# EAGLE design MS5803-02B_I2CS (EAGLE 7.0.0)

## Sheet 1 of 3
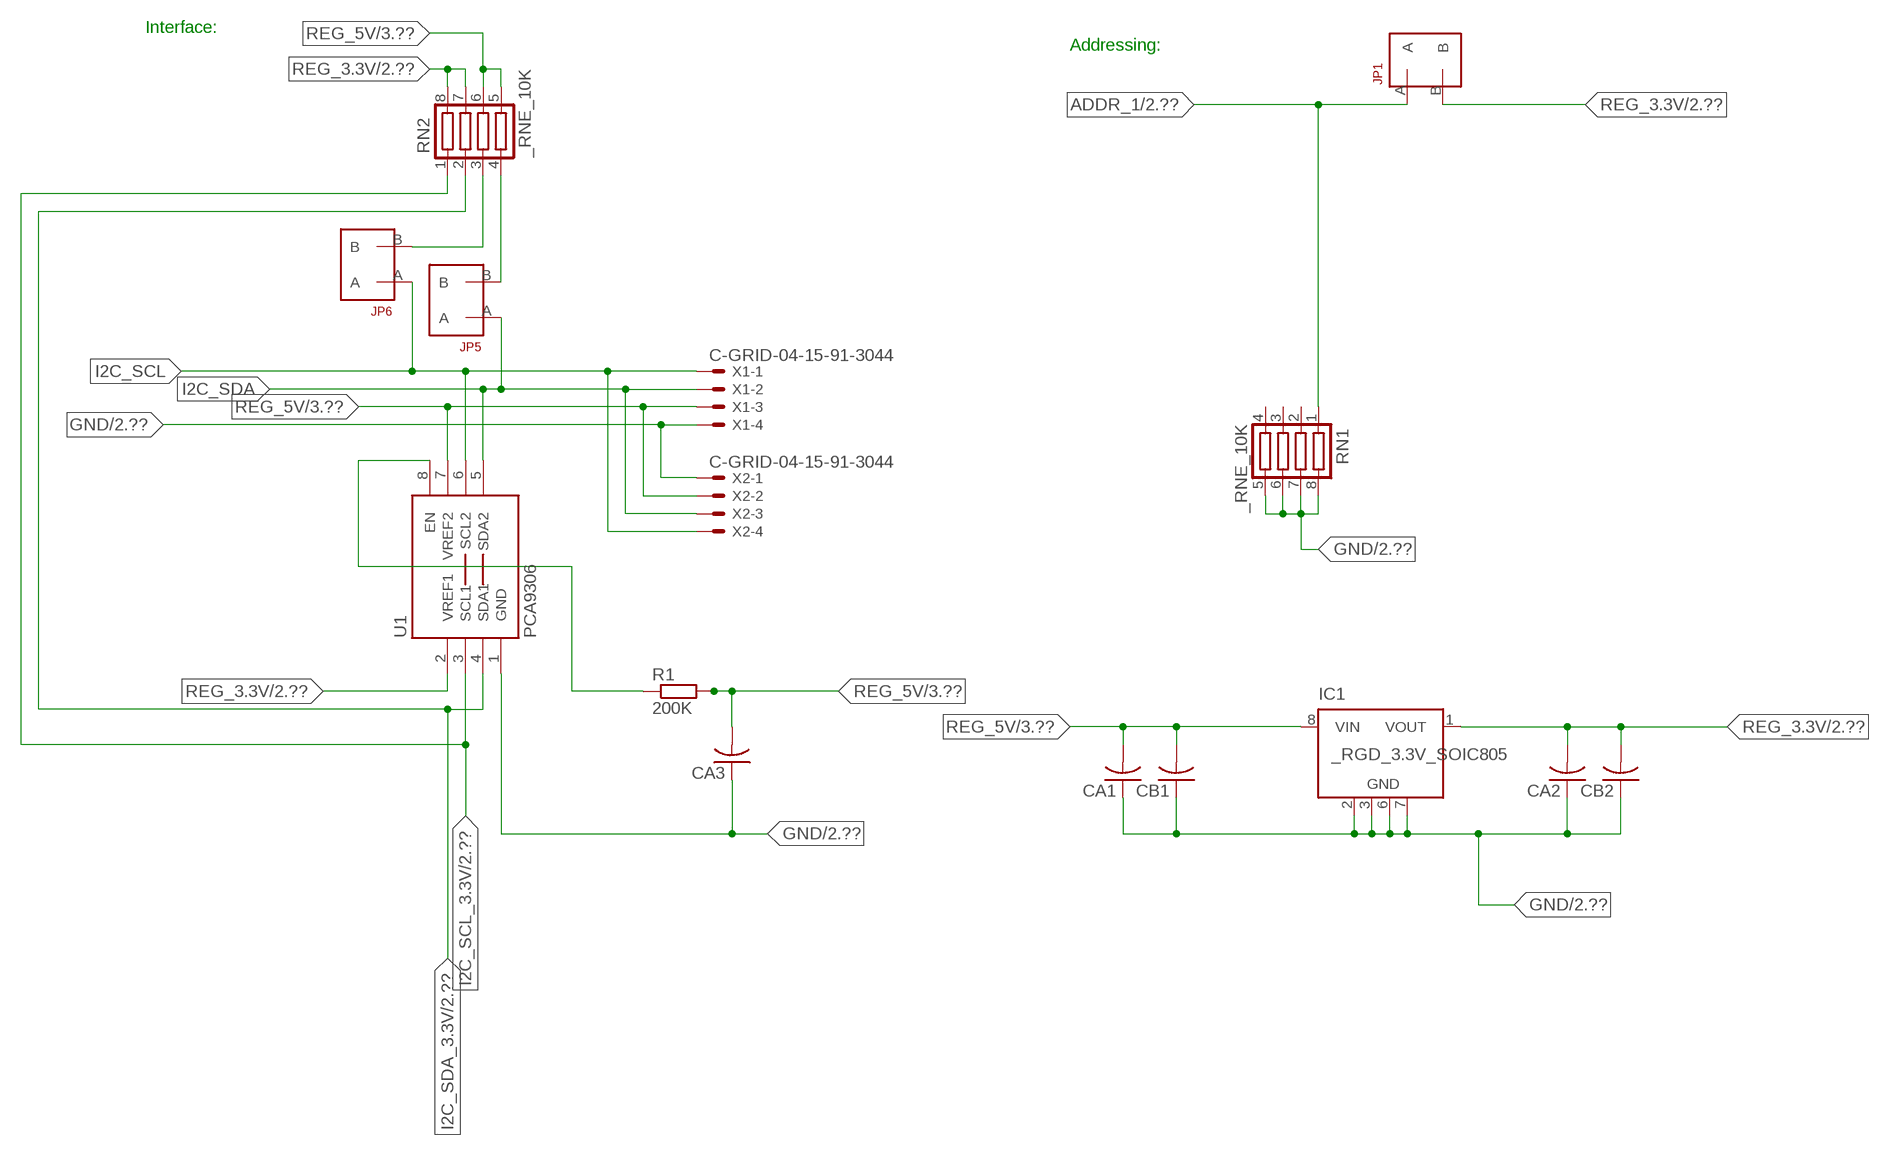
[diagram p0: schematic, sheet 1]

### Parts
CA1  CC1206KRX7R9BB104  [.1UF]
CA2  CC1206KRX7R9BB104  [.1UF]
CA3  CC1206KRX7R9BB104  [.1UF]
CB1  TMK316F106ZL-TC1206K  [TMK316F106ZL-T]
CB2  TMK316F106ZL-TC1206K  [TMK316F106ZL-T]
IC1  _RGD_3.3V_SOIC805  [_RGC_3.3V_SOIC8]
JP1  JUMPER_1X2_2MM  [JUMPER_1X2_2MM]
JP5  JUMPER_1X2_2MM  [JUMPER_1X2_2MM]
JP6  JUMPER_1X2_2MM  [JUMPER_1X2_2MM]
R1  200K  RESISTOR_SMT-0603  [R603]
RN1  _RNE_10K  [RNE]
RN2  _RNE_10K  [RNE]
U1  PCA9306  PCA9306_NCD  [PSOP-8]
X1  C-GRID-04-15-91-3044  [15-91-04]
X2  C-GRID-04-15-91-3044  [15-91-04]

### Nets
ADDR_1: JP1.A RN1.1 ; also sheet 2
GND: CA1.1 CA2.1 CA3.1 CB1.1 CB2.1 IC1.2(GND) IC1.3(GND) IC1.6(GND) IC1.7(GND) RN1.5 RN1.6 RN1.7 RN1.8 U1.1(GND) X1.4 X2.1 ; also sheet 2,3
I2C_SCL: JP6.A U1.6(SCL2) X1.1 X2.4
I2C_SCL_3.3V: RN2.1 U1.3(SCL1) ; also sheet 2
I2C_SDA: JP5.A U1.5(SDA2) X1.2 X2.3
I2C_SDA_3.3V: RN2.2 U1.4(SDA1) ; also sheet 2
N$1: JP6.B RN2.3
N$2: JP5.B RN2.4
N$24: R1.1 U1.8(EN)
REG_3.3V: CA2.2 CB2.2 IC1.1(VOUT) JP1.B RN2.7 RN2.8 U1.2(VREF1) ; also sheet 2
REG_5V: CA1.2 CA3.2 CB1.2 IC1.8(VIN) R1.2 RN2.5 RN2.6 U1.7(VREF2) X1.3 X2.2 ; also sheet 3
Unconnected: IC1.4(NC) IC1.5(NC) RN1.2 RN1.3 RN1.4

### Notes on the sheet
- Interface:
- Addressing:

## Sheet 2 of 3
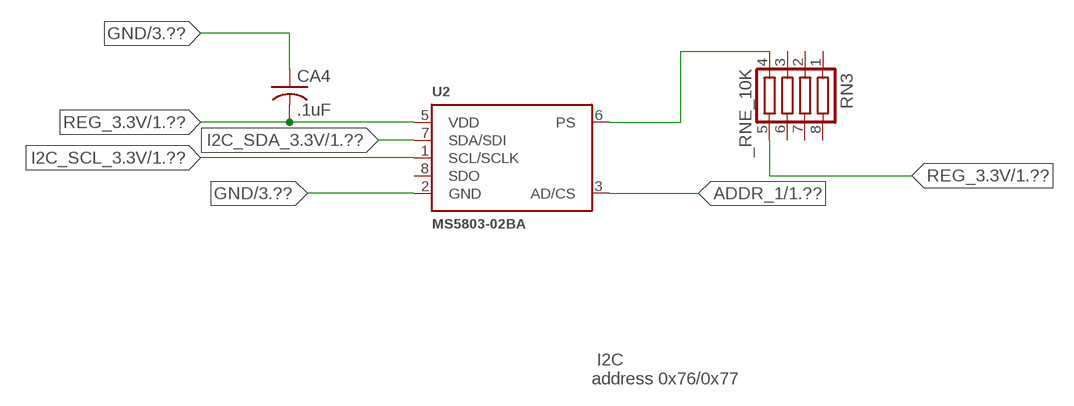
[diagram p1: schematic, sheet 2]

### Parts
CA4  .1uF  CC1206KRX7R9BB104C1206K  [CC1206KRX7R9BB104]
RN3  _RNE_10K  [RNE]
U2  MS5803-02BA  MS5803-14BA  [MS5803]

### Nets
ADDR_1: U2.3(AD/CS) ; also sheet 1
GND: CA4.1 U2.2(GND) ; also sheet 1,3
I2C_SCL_3.3V: U2.1(SCL/SCLK) ; also sheet 1
I2C_SDA_3.3V: U2.7(SDA/SDI) ; also sheet 1
N$4: RN3.4 U2.6(PS)
REG_3.3V: CA4.2 RN3.5 U2.5(VDD) ; also sheet 1
Unconnected: RN3.1 RN3.2 RN3.3 RN3.6 RN3.7 RN3.8 U2.8(SDO)

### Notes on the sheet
- I2C
  address 0x76/0x77

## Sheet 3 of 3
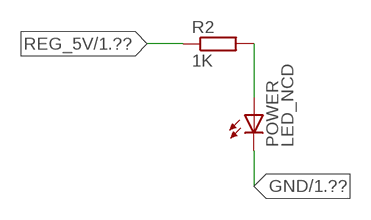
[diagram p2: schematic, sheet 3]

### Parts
POWER  LED_NCD  [CHIPLED_0603]
R2  1K  RESISTOR_SMT-0402  [R402]

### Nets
GND: POWER.C ; also sheet 1,2
N$5: POWER.A R2.2
REG_5V: R2.1 ; also sheet 1

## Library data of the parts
CA1-CA4 = NCD_ULTIMATE_LIBRARY:CC1206KRX7R9BB104: Capacitor CA .1uF 50V SMT C1206K CC1206KRX7R9BB104
CB1 CB2 = NCD_ULTIMATE_LIBRARY:TMK316F106ZL-T: Capacitor CB 10uF SMT 1206 TMK316F106ZL-T
IC1 = NCD_ULTIMATE_LIBRARY:_RGD_3.3V_SOIC8: Regulator Linear 3.3V Chip Positive VOLTAGE REGULATOR Digikey 497-1199-2-ND/L78L33ACD13TR
JP1 JP5 JP6 = NCD_ULTIMATE_CONNECTORS:JUMPER_1X2_2MM
POWER = NCD_ULTIMATE_LIBRARY:LED_NCD: LED Digikey 754-1132-2-ND/APT2012SRCPRV
R1 R2 = NCD_ULTIMATE_LIBRARY:RESISTOR_SMT: NCD Resistor
RN1-RN3 = NCD_ULTIMATE_LIBRARY:_RNE_10K: Resistor Array RNE SMT 10K x 4 Single Resistor Source: http://www.ctscorp.com/components/Datasheets/CTSChipArrayDs.pdf Digikey 742C083103JPTR-ND/742C083103JP; OC_FARNELL: unknown; OC_NEWARK: unknown
U1 = NCD_ULTIMATE_LIBRARY:PCA9306_NCD: NCD Bidirectional I2C level shifter. NOT compatible with all available part number pinout schemes- DOUBLE CHECK!!!; PROD_ID: IC-10023
U2 = MS5803:MS5803-14BA; PROD_ID: IC-12111
X1 X2 = NCD_ULTIMATE_CONNECTORS:C-GRID-04: CONNECTOR 4-Pos I2C wire to board 2.54 mm (0.100") pitch header Digikey WM1342-ND/0015912045; OC_FARNELL: unknown; OC_NEWARK: unknown

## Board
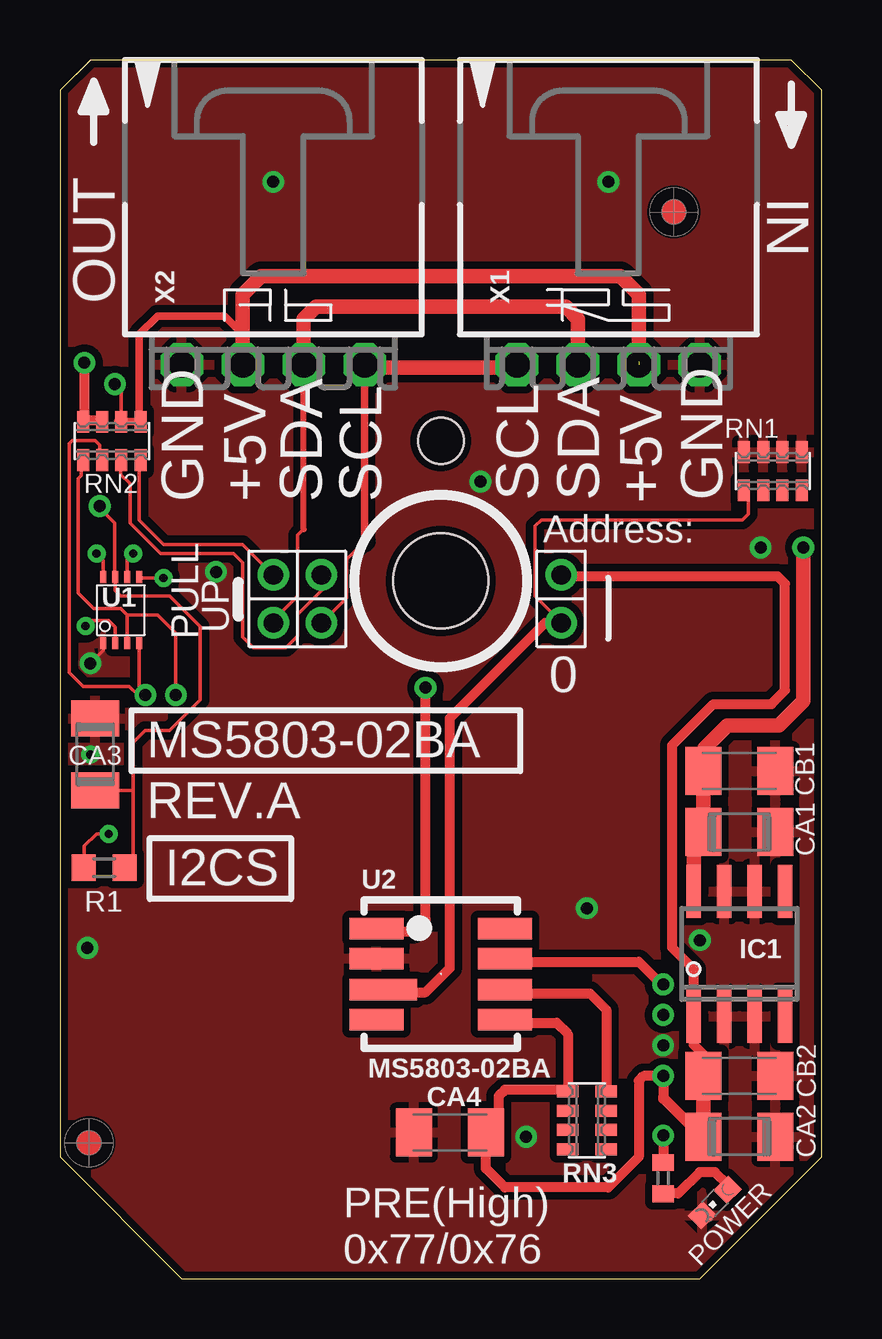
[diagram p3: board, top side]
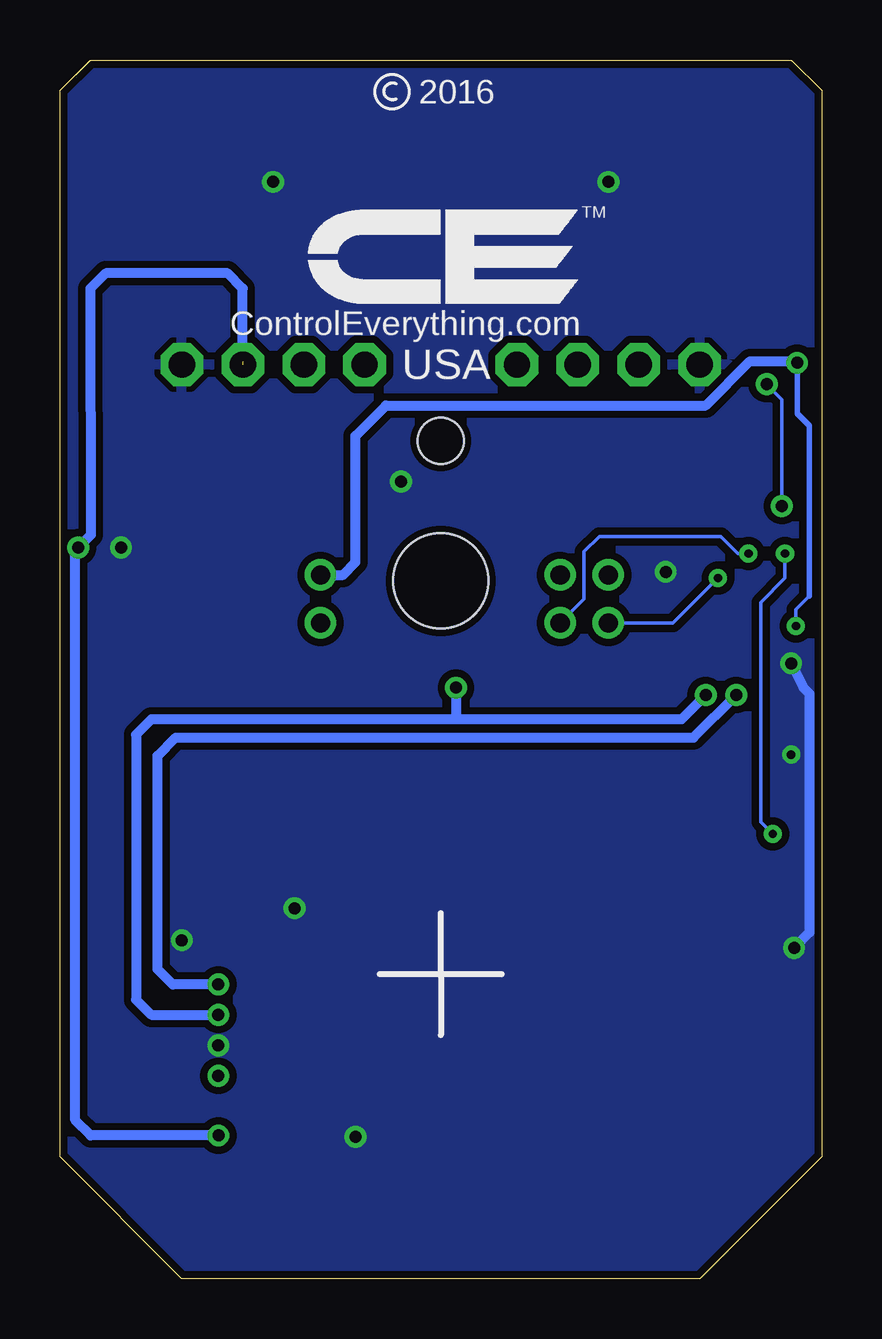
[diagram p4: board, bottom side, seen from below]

Size 31.75 x 50.8 mm. Coordinates in mm from the lower left corner, seen from the top.
Outline: 32 segments
Copper layers (1*16): Top 0.035mm / dielectric 1.5mm / Bottom 0.035mm
Design rules "default": minimum track width 5mil, minimum drill 24mil, track to track 5mil, track to pad 5mil, pad to pad 5mil, via to via 5mil, smd to smd 5mil, copper to edge 10mil, drill to drill 8mil, minimum pad ring 10mil, minimum via ring 8mil, stop-mask expansion 2mil, vias tented up to drill 0mil, thermal gap 10mil
Holes 3.96 mm at 15.88,29.08
Holes 1.91 mm at 15.88,34.93

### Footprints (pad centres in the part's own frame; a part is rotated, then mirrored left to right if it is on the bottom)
.1UF = smd 1.5 x 2: 1 -1.5,0; 2 1.5,0
CC1206KRX7R9BB104 = smd 1.5 x 2: 1 -1.5,0; 2 1.5,0
TMK316F106ZL-T = smd 1.5 x 2: 1 -1.5,0; 2 1.5,0
_RGC_3.3V_SOIC8 = smd 0.6 x 2.2: 1 -1.905,-2.6; 2 -0.635,-2.6; 3 0.635,-2.6; 4 1.905,-2.6; 5 1.905,2.6; 6 0.635,2.6; 7 -0.635,2.6; 8 -1.905,2.6
JUMPER_1X2_2MM = drill 0.8: A 0,2; B 0,0
CHIPLED_0603 = smd 0.8 x 0.876: A 0,-0.75; C 0,0.75
R603 = smd 1 x 1.1: 1 -0.85,0; 2 0.85,0
R402 = smd 0.7 x 0.9: 1 -0.65,0; 2 0.65,0
RNE = smd 0.5 x 0.9: 1 -1.2,-0.8; 2 -0.4,-0.8; 3 0.4,-0.8; 4 1.2,-0.8; 5 1.2,0.8; 6 0.4,0.8; 7 -0.4,0.8; 8 -1.2,0.8
PSOP-8 = smd 0.25 x 0.5: 1 -0.73,-1.37; 2 -0.23,-1.37; 3 0.27,-1.37; 4 0.77,-1.37; 5 0.77,1.38; 6 0.27,1.38; 7 -0.23,1.38; 8 -0.73,1.38
MS5803 = smd 2.25 x 0.9: 1 -2.675,1.9; 2 -2.675,0.65; 4 -2.675,-1.9; 5 2.675,-1.9; 6 2.675,-0.65; 7 2.675,0.65; 8 2.675,1.9 | smd 2.8 x 0.9: 3 -2.4,-0.65
15-91-04 = drill 1.1 pad 1.778 octagon: 1 -3.81,-7.62; 2 -1.27,-7.62; 3 1.27,-7.62; 4 3.81,-7.62

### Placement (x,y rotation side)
CA1  28.32,18.62 180 top
CA2  28.32,5.92 180 top
CA3  1.46,21.86 270 top
CA4  16.26,6.1 0 top
CB1  28.32,21.16 180 top
CB2  28.32,8.46 180 top
IC1  28.32,13.54 0 top
JP1  20.89,29.34 180 top
JP5  8.89,29.34 180 top
JP6  10.9,29.34 180 top
POWER  27.3,3.18 135 top
R1  1.84,17.13 0 top
R2  25.15,4.19 270 top
RN1  29.72,33.66 0 top
RN2  2.16,34.93 0 top
RN3  21.97,6.6 90 top
U1  2.54,27.86 0 top
U2  15.88,12.7 0 top
U$5  [VISION_REF10]  1.21,5.66 90 top
U$28  [VISION_REF10]  25.59,44.46 90 top
X1  22.86,45.72 0 top
X2  8.89,45.72 0 top

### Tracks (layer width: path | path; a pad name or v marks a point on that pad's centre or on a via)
ADDR_1
  Top 0.152: JP1.A 20.89,27.37 19.81,28.45 19.81,31.37 20.07,31.62 28.45,31.62 28.7,31.88 28.7,32.78 RN1.1
  Top 0.406: U2.3 13.71,11.94 15.24,11.94 16.26,12.95 16.26,23.37 20.23,27.34 JP1.A
GND  (via drill 0.35, 0.5)
  Top 0.152: CA3.1 1.52,23.42 1.52,23.62 | v1.27,25.65 1.81,26.19 U1.1
  Bottom 0.406: v1.27,25.65 0.76,24.64 0.51,24.38 0.51,14.43 v1.15,13.79
  other vias: 8.89,45.72 22.86,45.72 25.15,9.73 17.53,33.22 26.67,14.11 6.5,29.46 29.21,30.48 21.97,15.44 19.43,5.92 1.27,21.84
  pour Bottom (isolate 0.305): -0.64,5.08 -0.64,49.53 1.27,51.44 30.48,51.44 32.38,49.53 32.38,5.08 26.67,-0.63 5.08,-0.63
  pour Top (isolate 0.305): 4.45,-1.27 -1.27,4.45 -1.27,50.17 0.64,52.07 31.11,52.07 33.02,50.17 33.02,4.45 27.3,-1.27
I2C_SCL  (via drill 0.35)
  Top 0.152: 12.7,30.73 11.94,29.97 11.94,28.38 JP6.A | v3.05,30.23 2.81,29.99 U1.6
  Top 0.305: 12.7,30.73 X2.4
  Top 0.406: X2.4 12.7,37.97 | 19.05,37.97 X1.1
  Top 0.61: 12.7,37.97 19.05,37.97
  Bottom 0.152: JP6.A 9.91,28.33 9.91,30.3 9.27,30.94 4.19,30.94 3.48,30.23 v3.05,30.23
I2C_SCL_3.3V  (via drill 0.5)
  Top 0.152: RN2.1 0.89,34.07 0.89,33.48 0.77,33.35 0.77,28.59 1.41,27.94 2.54,27.94 2.81,27.67 | 2.81,27.67 U1.3 | v4.83,24.33 v4.83,24.34 4.83,26.92 4.08,27.67 2.81,27.67
  Top 0.406: U2.1 13.45,14.48 14.73,14.48 15.24,14.99 v15.24,24.64
  Bottom 0.406: v4.83,24.33 5.84,23.32 15.24,23.32 | 15.24,23.32 27.94,23.32 28.58,22.68 28.58,11.63 27.94,11 v25.15,11 | v15.24,24.64 15.24,23.32
I2C_SDA  (via drill 0.35)
  Top 0.152: JP5.A 8.89,27.44 9.91,28.45 9.91,30.99 10.16,31.24 | U1.5 3.34,29.21 v4.32,29.21
  Top 0.254: 10.16,31.24 10.16,31.25 X2.3
  Top 0.61: X2.3 10.16,40.01 10.67,40.51 21.09,40.51 21.59,40.01 X1.2
  Bottom 0.152: v4.32,29.21 6.19,27.34 JP5.A
I2C_SDA_3.3V  (via drill 0.5)
  Top 0.152: RN2.2 1.65,34.14 1.65,34.75 1.46,34.94 0.51,34.94 0.38,34.81 0.38,26.37 0.38,26.36 0.38,25.27 0.96,24.69 2.9,24.69 3.25,24.33 v3.56,24.33 3.31,24.58 U1.4
  Top 0.406: U2.7 18.82,13.21 24.13,13.21 25.07,12.27 v25.15,12.27
  Bottom 0.406: v25.15,12.27 27.05,12.27 27.69,12.9 27.69,21.79 26.93,22.56 5.34,22.56 v3.56,24.33
N$1
  Top 0.152: JP6.B 10.92,29.31 10.92,28.7 9.91,27.69 9.91,26.8 9.42,26.31 8.06,26.31 7.62,26.75 7.62,29.84 7.24,30.23 4.19,30.23 2.92,31.5 2.92,33.15 2.54,33.53 2.54,34.1 RN2.3
  Top 0.305: 2.54,34.02 RN2.3
N$2
  Top 0.152: JP5.B 7.62,30.61 4.32,30.61 3.3,31.62 3.3,34.07 RN2.4
  Top 0.305: 3.37,33.88 RN2.4
N$4
  Top 0.406: U2.6 18.84,11.89 22.1,11.89 22.77,11.21 RN3.4
N$5
  Top 0.406: POWER.A 27.84,3.92 27.3,4.45 26.67,4.45 25.78,3.56 25.16,3.56 R2.2
N$24  (via drill 0.35)
  Top 0.152: R1.1 1.02,17.16 1.02,18.03 1.52,18.54 v2.03,18.54 | v1.52,30.23 1.81,29.94 U1.8
  Bottom 0.152: v2.03,18.54 2.54,19.05 2.54,28.19 1.52,29.21 v1.52,30.23
REG_3.3V  (via drill 0.35, 0.5)
  Top 0.152: v1.07,27.2 1.27,27.43 2.03,27.43 2.31,27.16 U1.2
  Top 0.406: CB2.2 26.82,9.35 26.42,9.75 26.42,10.36 | 26.82,6.55 26.16,6.55 25.15,7.57 v25.15,8.46 | IC1.1 26.42,12.9 25.53,13.79 25.53,22.24 27.24,23.95 29.66,23.95 30.23,24.52 30.23,28.97 29.91,29.29 20.95,29.29 JP1.B | 26.52,5.62 CA2.2 | v1.02,38.18 1.02,35.78 | 1.02,35.78 RN2.8 | 1.02,35.78 1.71,35.78 RN2.7 | v25.15,8.46 25.15,7.49 26.54,6.1 27.18,6.1 26.92,5.84 | U2.5 18.8,10.92 19.05,10.67 20.7,10.67 21.17,10.2 RN3.5 21.36,7.87 18.54,7.87 18.29,7.62 18.29,6.6 17.78,6.1 CA4.2 17.76,4.6 18.54,3.81 22.86,3.81 24.13,5.08 24.13,8.26 24.33,8.46 v25.15,8.46
  Top 0.61: CB2.2 26.82,6.55 CA2.2 | 26.42,10.36 IC1.1
  Bottom 0.152: 0.51,28.45 1.07,27.89 v1.07,27.2
  Bottom 0.229: 0.51,28.45 0.51,35.56 1.02,36.07 v1.02,38.18
  Bottom 0.406: v1.02,38.18 1.08,38.24 2.99,38.24 4.83,36.4 18.16,36.4 19.43,35.13 19.43,29.87 19.94,29.34 JP1.B
REG_5V  (via drill 0.5)  (1 unrouted)
  Top 0.152: RN2.6 2.56,37.01 v2.29,37.29 | R1.2 3.05,17.49 3.05,20.36 | 3.05,20.36 3.05,22.35 3.56,22.86 4.57,22.86 5.84,24.13 5.84,27.18 4.57,28.45 2.54,28.45 2.31,28.68 U1.7 2.29,29.27 2.29,31.5 1.65,32.13 v1.65,32.21 | CA3.2 3.05,20.36
  Top 0.305: 7.62,39.37 7.5,39.37 | 2.42,35.74 RN2.6 RN2.5 3.31,35.8 3.31,39.37 4.07,40.13 6.86,40.13 7.62,39.37 | X2.2 7.62,39.37
  Top 0.406: v25.15,5.97 R2.1
  Top 0.61: X2.2 7.62,41.02 8.38,41.78 23.37,41.78 24.13,41.02 24.13,38.23 | IC1.8 26.42,18.21 CA1.2 CB1.2 26.86,21.2 26.86,22.11 27.82,23.06 29.98,23.06 30.99,24.08 v30.99,30.48
  Bottom 0.152: v1.65,32.21 1.65,36.65 v2.29,37.29
  Bottom 0.406: X1.3 24.13,41.28 24.77,41.91 29.84,41.91 30.48,41.27 30.47,31 v30.99,30.48 31.11,30.36 31.11,6.6 30.48,5.97 v25.15,5.97

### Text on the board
tNames: IN | OUT | GND | +5V | SDA | SCL | SCL | SDA | +5V | GND | Address: | PULL | UP | 0 | MS5803-02BA | REV.A | I2CS | PRE(High) / 0x77/0x76
bNames: 2016 | TM | ControlEverything.com | USA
